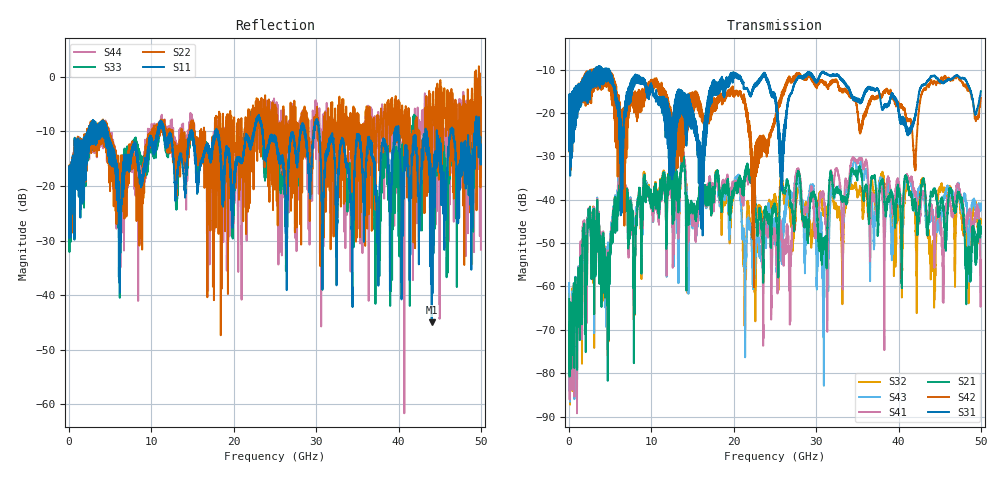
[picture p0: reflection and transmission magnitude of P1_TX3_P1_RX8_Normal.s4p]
!Keysight Technologies,N5225B,MY57041031,A.13.20.10
!Date: Friday, May 31, 2019 11:25:48
!Correction: S11(Full 4 Port(1,2,3,4))
!S12(Full 4 Port(1,2,3,4))
!S13(Full 4 Port(1,2,3,4))
!S14(Full 4 Port(1,2,3,4))
!S21(Full 4 Port(1,2,3,4))
!S22(Full 4 Port(1,2,3,4))
!S23(Full 4 Port(1,2,3,4))
!S24(Full 4 Port(1,2,3,4))
!S31(Full 4 Port(1,2,3,4))
!S32(Full 4 Port(1,2,3,4))
!S33(Full 4 Port(1,2,3,4))
!S34(Full 4 Port(1,2,3,4))
!S41(Full 4 Port(1,2,3,4))
!S42(Full 4 Port(1,2,3,4))
!S43(Full 4 Port(1,2,3,4))
!S44(Full 4 Port(1,2,3,4))
!S4P File: Measurements: <S11,S12,S13,S14>,
!<S21,S22,S23,S24>,
!<S31,S32,S33,S34>,
!<S41,S42,S43,S44>:
# Hz S  dB  R 50.0
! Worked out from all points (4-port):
!   5000 points, 10 MHz to 50 GHz, reference 50 ohm
!   strongest paths, dB at 10 MHz, 12.51 GHz, 25.01 GHz, 37.51 GHz, 50 GHz:
!     S31: -19.4, -27.1, -15.7, -14.5, -15.0
!     S42: -19.4, -24.4, -22.2, -16.4, -16.5
!     S21: -62.9, -35.7, -41.7, -47.2, -47.5
!     S41: -75.6, -37.1, -48.0, -42.2, -61.3
!     S43: -59.2, -36.5, -46.7, -38.6, -41.9
!     S32: -65.2, -35.2, -39.2, -41.0, -44.7
!   lowest |S11| = -45.0 dB at 44.03 GHz (marker M1), VSWR 1.01, Z = 49.8 + j0.512 ohm
!   |S11| at or under -10 dB: 4.66 GHz to 10.77 GHz (6.106 GHz wide, 79.2 % of centre); 23.49 GHz to 28.08 GHz (4.583 GHz wide, 17.8 % of centre); 30.37 GHz to 39.61 GHz (9.238 GHz wide, 26.4 % of centre)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
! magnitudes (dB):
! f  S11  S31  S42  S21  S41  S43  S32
! 10 MHz  -19.5  -19.4  -19.4  -62.9  -75.6  -59.2  -65.2
! 6.37 GHz  -23.4  -27.2  -21.3  -34.3  -33.2  -32.2  -33.1
! 20.62 GHz  -15.0  -11.8  -15.3  -36.0  -36.3  -35.1  -35.2
! 22.44 GHz  -9.8  -13.9  -32.8  -35.6  -35.9  -57.2  -53.9
! 37.97 GHz  -12.6  -18.8  -16.4  -35.9  -37.7  -35.4  -34.7
! 44.03 GHz  -45.0  -11.4  -12.7  -38.7  -41.5  -44.1  -52.5
! 50 GHz  -12.4  -15.0  -16.5  -47.5  -61.3  -41.9  -44.7
